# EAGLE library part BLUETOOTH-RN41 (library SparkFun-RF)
Bluetooth SMD module
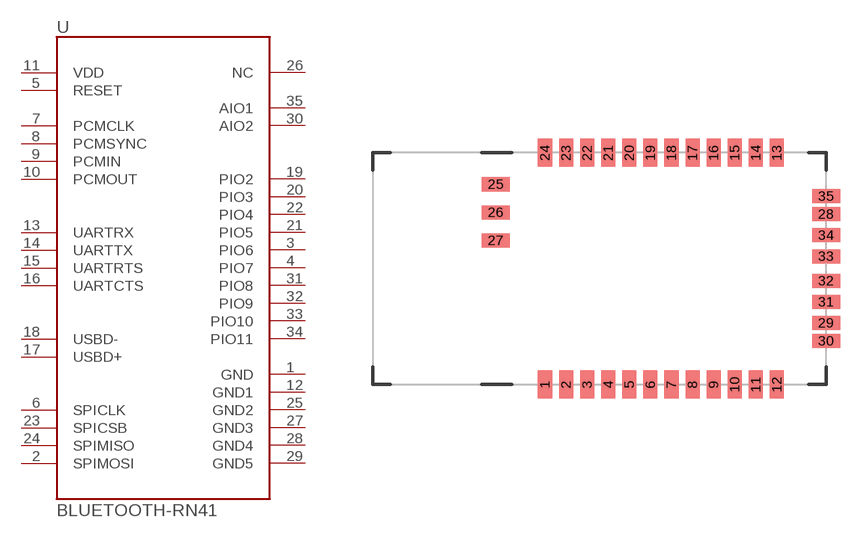
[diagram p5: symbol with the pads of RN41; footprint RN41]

Designator prefix -

## BLUETOOTH-RN41"  [RN41]
1  GND
2  SPIMOSI
3  PIO6
4  PIO7
5  RESET
6  SPICLK
7  PCMCLK
8  PCMSYNC
9  PCMIN
10  PCMOUT
11  VDD
12  GND1
13  UARTRX
14  UARTTX
15  UARTRTS
16  UARTCTS
17  USBD+
18  USBD-
19  PIO2
20  PIO3
21  PIO5
22  PIO4
23  SPICSB
24  SPIMISO
25  GND2
26  NC
27  GND3
28  GND4
29  GND5
30  AIO2
31  PIO8
32  PIO9
33  PIO10
34  PIO11
35  AIO1

## Footprint RN41 (pad centres in mm)
smd 0.8 x 1.6: 1 -6.6,-6.6; 2 -5.4,-6.6; 3 -4.2,-6.6; 4 -3,-6.6; 5 -1.8,-6.6; 6 -0.6,-6.6; 7 0.6,-6.6; 8 1.8,-6.6; 9 3,-6.6; 10 4.2,-6.6; 11 5.4,-6.6; 12 6.6,-6.6; 13 6.6,6.6; 14 5.4,6.6; 15 4.2,6.6; 16 3,6.6; 17 1.8,6.6; 18 0.6,6.6; 19 -0.6,6.6; 20 -1.8,6.6; 21 -3,6.6; 22 -4.2,6.6; 23 -5.4,6.6; 24 -6.6,6.6
smd 1.6 x 0.8: 25 -9.4,4.8; 26 -9.4,3.2; 27 -9.4,1.6; 28 9.4,3.1; 29 9.4,-3.1; 30 9.4,-4.122; 31 9.4,-1.9; 32 9.4,-0.7; 33 9.4,0.7; 34 9.4,1.9; 35 9.4,4.122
